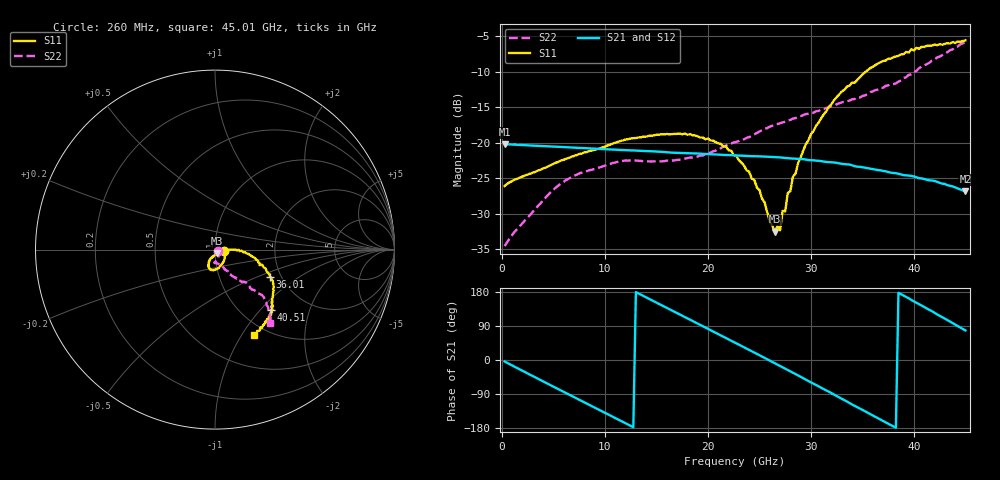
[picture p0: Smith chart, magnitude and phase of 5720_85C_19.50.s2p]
! Device:  ADRF5720
! Description: 0.5dB LSB GaAs MMIC 6-bit Digital Attenuator
! Frequency:  0.000009 -  40 GHz
! Ports:
!	RF1	= Port 1
!	RF2	= Port 2
! Vdd:  3.3 Volt
! Vss:  -3.3 Volt
! Control:  0/3.3 Volt
! State:  19.50 dB attenuation
! Data:  The device was measured using G-S-G Probes on a matrix board.
!  Data was collected using an calibrated 4 port network analyzer.
!  The reference plane for this measurement is at the launchers.
! Note:  Analog Devices supplies this data as a sample of measured data
!  for this product.  Your particular data for this product may vary.
!  Data was taken at 85 degrees C.
!  Analog Devices reserves the right to change this data at anytime.
# GHZ S DB R 45.0
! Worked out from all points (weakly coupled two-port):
!   180 points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, 260 MHz to 45.01 GHz, reference 45 ohm
!   highest |S21| = -20.22 dB at 260 MHz (marker M1); lowest = -26.9 dB at 45.01 GHz (marker M2)
!   lowest |S11| = -32.5 dB at 26.51 GHz (marker M3), VSWR 1.05, Z = 45.9 - j1.95 ohm
!   |S11| at or under -10 dB: start of sweep to 35.35 GHz
!   |S22| runs from -34.6 to -5.8 dB; largest |S21 - S12| = 0.00049
!   S11 on the Smith chart (normalised r, x): 260 MHz: 1.10, -0.02; 36.01 GHz: 1.75, -0.60; 40.51 GHz: 1.34, -1.14; 45.01 GHz: 0.87, -1.14
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0.26  -26.11 -10.5  -20.22 -3.9  -20.22 -3.9  -34.58 -25.8
4.76  -23.17 -38.2  -20.55 -67.0  -20.53 -66.9  -26.95 -65.2
7.76  -21.54 -57.3  -20.76 -108.4  -20.75 -108.3  -24.22 -81.3
11.51  -19.78 -77.2  -21.03 -160.1  -21.03 -160.0  -22.61 -92.5
15.26  -18.91 -92.5  -21.28 147.9  -21.27 148.0  -22.63 -91.2
20.01  -19.42 -108.7  -21.62 82.2  -21.60 82.4  -21.54 -75.0
22.76  -21.87 -114.5  -21.81 44.0  -21.80 44.2  -19.90 -67.0
25.01  -26.68 -108.4  -21.94 12.6  -21.93 12.9  -18.45 -64.0
26.51  -32.53 -63.7  -22.06 -8.7  -22.04 -8.4  -17.45 -60.9
26.76  -31.75 -50.2  -22.07 -12.3  -22.06 -12.0  -17.39 -60.8
27.01  -32.35 -36.1  -22.09 -15.9  -22.07 -15.6  -17.28 -60.0
27.26  -29.61 -24.5  -22.13 -19.5  -22.12 -19.2  -17.16 -60.4
27.51  -29.68 -15.9  -22.17 -23.0  -22.15 -22.7  -17.08 -59.4
27.76  -27.10 -11.0  -22.19 -26.5  -22.18 -26.3  -16.88 -60.1
28.01  -26.84 -7.7  -22.23 -30.1  -22.22 -29.9  -16.81 -59.5
28.26  -24.79 -4.4  -22.25 -33.6  -22.24 -33.3  -16.63 -60.0
30.26  -18.36 -2.0  -22.50 -62.3  -22.49 -62.1  -15.81 -58.2
33.01  -12.81 -12.2  -23.00 -102.5  -22.99 -102.2  -14.34 -54.6
36.01  -9.35 -26.2  -23.73 -146.2  -23.71 -146.0  -12.80 -50.7
37.76  -8.19 -33.5  -24.23 -171.7  -24.22 -171.3  -11.79 -47.0
40.51  -6.79 -47.4  -25.02 147.2  -25.00 147.7  -9.52 -44.9
45.01  -5.63 -65.2  -26.88 78.0  -26.85 78.4  -5.82 -52.8
